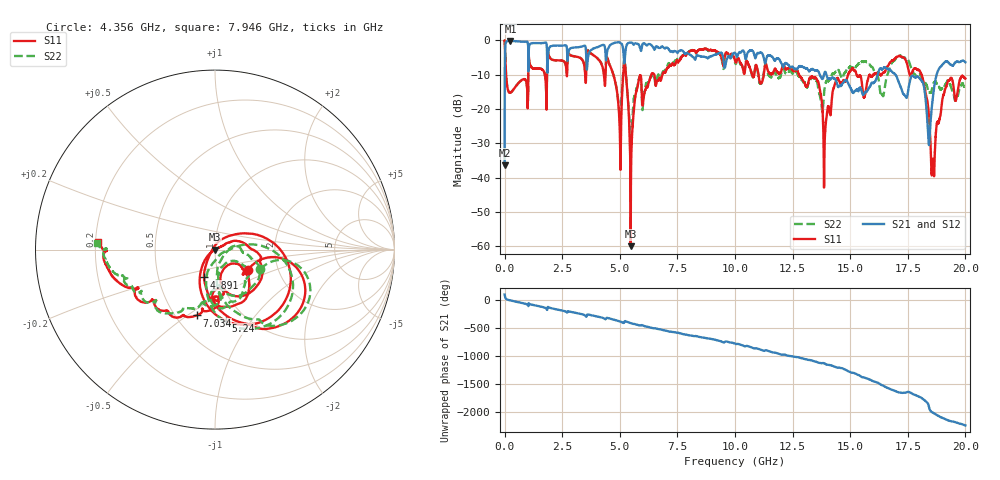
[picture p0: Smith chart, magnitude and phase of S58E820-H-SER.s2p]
!{S58E820}
!Johanson Technology Inc.
!www.johansontechnology.com
!Test Board Conditions:
!Substrate Type  RO4350B
!Substrate Thickness  60 mil
!Substrate Dk  3.66
!TL Type: GCPW
!TL Trace Width  115 mil
!TL Gap  52 mil
!Electrode orientation  Horizontal
!DUT TOPOLOGY	SERIES
!Mounting Pad LxW  55x428 mil
! Created Wed Apr 14 12:04:06 2021
# mhz S ma R 50
! 2 Port Network Data from SP1.SP block
! freq  magS11  angS11  magS21  angS21  magS12  angS12  magS22  angS22
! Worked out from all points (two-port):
!   20001 points, 300 kHz to 20 GHz, reference 50 ohm
!   highest |S21| = -0.14 dB at 251.3 MHz (marker M1); lowest = -36.4 dB at 300 kHz (marker M2)
!   |S21| within 3 dB of the highest: 19.47 MHz to 1.027 GHz (1.007 GHz wide, 193 % of centre); 5.245 GHz to 7.176 GHz (1.931 GHz wide, 31.1 % of centre)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
!   lowest |S11| = -60.0 dB at 5.473 GHz (marker M3), VSWR 1.00, Z = 50 - j0.0998 ohm
!   |S11| at or under -10 dB: 5.267 GHz to 6.374 GHz (1.107 GHz wide, 19 % of centre); 12.77 GHz to 14.91 GHz (2.136 GHz wide, 15.4 % of centre); 18.1 GHz to end of sweep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
!   |S22| runs from -28.2 to 0.0 dB; largest |S21 - S12| = 0.012
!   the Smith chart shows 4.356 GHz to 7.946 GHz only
!   S11 on the Smith chart (normalised r, x): 4.356 GHz: 1.41, -0.33; 4.891 GHz: 0.85, -0.27; 5.24 GHz: 0.81, -0.76; 7.034 GHz: 0.63, -0.54; 7.946 GHz: 0.21, +0.03
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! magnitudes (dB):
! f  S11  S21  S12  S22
! 300 kHz  0.0  -36.4  -36.4  -0.1
! 104.3 MHz  -13.0  -0.2  -0.2  -12.9
! 251.3 MHz  -15.2  -0.1  -0.2  -15.2
! 3.334 GHz  -5.4  -1.8  -1.8  -5.3
! 4.356 GHz  -13.3  -2.1  -2.1  -11.2
! 4.891 GHz  -15.5  -0.5  -0.5  -15.2
! 5.24 GHz  -7.9  -3.4  -3.4  -7.5
! 5.473 GHz  -60.0  -0.6  -0.6  -27.8
! 5.829 GHz  -11.4  -1.3  -1.3  -11.3
! 6.667 GHz  -11.7  -2.1  -2.1  -10.0
! 7.034 GHz  -8.4  -2.1  -2.1  -7.9
! 7.946 GHz  -3.7  -3.8  -3.7  -3.6
! 10 GHz  -5.8  -3.7  -3.7  -6.3
! 13.33 GHz  -10.6  -8.4  -8.4  -10.6
! 13.91 GHz  -27.5  -9.2  -9.1  -13.2
! 14.42 GHz  -11.3  -12.3  -12.3  -8.9
! 16.67 GHz  -7.1  -8.4  -8.5  -9.0
! 18.07 GHz  -9.5  -11.5  -11.5  -10.1
! 18.41 GHz  -21.3  -30.2  -30.2  -15.1
! 18.59 GHz  -35.1  -16.7  -16.7  -13.1
! 19.19 GHz  -13.1  -6.1  -6.2  -12.3
! 20 GHz  -11.2  -6.4  -6.3  -13.7
